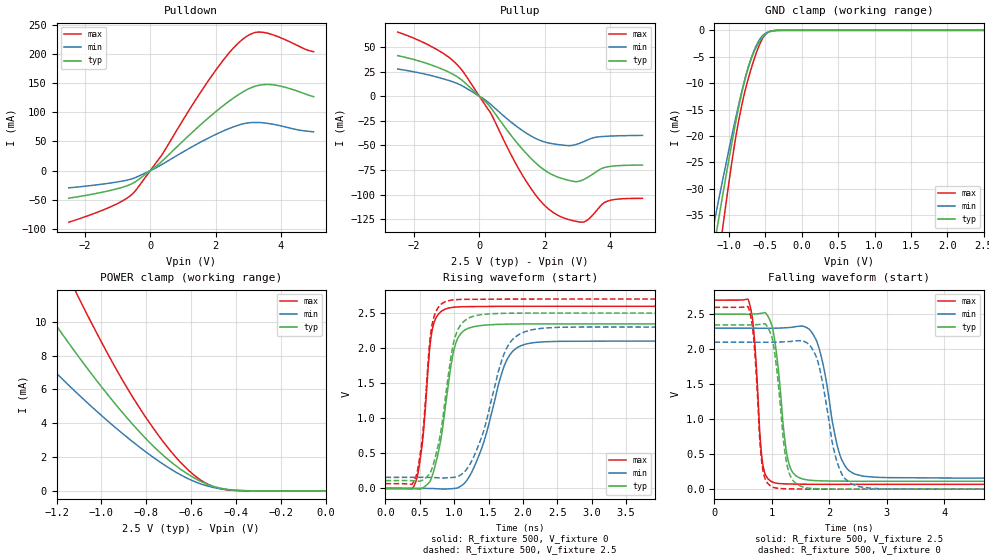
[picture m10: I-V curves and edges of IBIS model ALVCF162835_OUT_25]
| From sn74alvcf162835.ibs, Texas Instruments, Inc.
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[Model]   ALVCF162835_OUT_25
Model_type  3-state
Enable   Active-Low
Vref =   0
Rref =   500
Cref =   30p
Vmeas =   1.25
| variable   typ   min   max
C_comp   2.98pF   2.69pF   3.33pF
| C_pullup   3.41pF   2.52pF   4.48pF
| C_pulldown   2.44pF   2.04pF   2.92pF
| C_tri-state   2.98pF   2.69pF   3.33pF
[Temperature Range]   40   100   -40
| Ambient temperature   25   85   -40
[Voltage range]   2.5   2.3   2.7
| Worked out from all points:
|   slope of the pulldown table from 0 to 0.375 V, typ, clamps not added: 22 ohm
|   slope of the pullup table from 0 to 0.375 V, typ, clamps not added: 29.3 ohm
|   GND clamp passes 1 mA (typ) near -0.52 V on its own axis
|   POWER clamp passes 1 mA (typ) near -0.62 V on its own axis
|   rising waveform, R_fixture 500, V_fixture 0: 20-80 % time 217ps typ, 366ps min, 133ps max; typ from 0 V to 2.35 V
|   falling waveform, R_fixture 500, V_fixture 2.5: 20-80 % time 177ps typ, 283ps min, 116ps max; typ from 2.5 V to 0.112 V
|   rising waveform, R_fixture 500, V_fixture 2.5: 20-80 % time 219ps typ, 366ps min, 134ps max; typ from 0.112 V to 2.5 V
|   falling waveform, R_fixture 500, V_fixture 0: 20-80 % time 177ps typ, 281ps min, 117ps max; typ from 2.35 V to 0 V
[GND Clamp]
| ALVCF162835_OUT_25
|   Voltage   I(typ)   I(min)   I(max)
-2.5V     -156.5mA   -133.7mA   -196.4mA
-1.22V    -42.15mA   -37.53mA   -51.39mA
-1.16V    -37.17mA   -33.34mA   -45.01mA
-1.08V    -30.65mA   -27.85mA   -36.68mA
-925mV    -18.66mA   -17.64mA   -21.71mA
-800mV    -10.4mA    -10.2mA    -12.64mA
-715mV    -6.256mA   -6.058mA   -8.169mA
-645mV    -3.755mA   -3.482mA   -5.072mA
-560mV    -1.73mA    -1.371mA   -2.101mA
-485mV    -620.5uA   -458.2uA   -582.7uA
-295mV    -6.427uA   -8.451uA   -1.684uA
2.5V      1.046nA    413.3nA    70.04pA
[POWER Clamp]
| ALVCF162835_OUT_25
|   Voltage   I(typ)   I(min)   I(max)
-2.5V     39.5mA     27.67mA    55.72mA
-1.515V   16.12mA    11.35mA    23.37mA
-1.28V    11.3mA     8.018mA    16.39mA
-1.115V   8.181mA    5.861mA    11.8mA
-1.095V   7.82mA     5.611mA    11.26mA
-935mV    5.092mA    3.717mA    7.225mA
-810mV    3.206mA    2.388mA    4.506mA
-690mV    1.714mA    1.285mA    2.335mA
-575mV    685.4uA    501.9uA    806.4uA
-505mV    287.7uA    216.5uA    272.5uA
-430mV    75.11uA    63.49uA    49.86uA
-31.15fV  1.046nA    2.588nA    84.19pA
[Pulldown]
| ALVCF162835_OUT_25
|   Voltage   I(typ)   I(min)   I(max)
-2.5V     -47.43mA   -29.66mA   -88.64mA
-1.18V    -33.52mA   -21.01mA   -61.26mA
-515mV    -21.1mA    -13.25mA   -38.15mA
355mV     16mA       10.5mA     27.2mA
1.3V      66.49mA    41.5mA     113.8mA
1.985V    100.3mA    61.58mA    170.9mA
2.49V     122.4mA    73.87mA    207.1mA
2.915V    137.7mA    81.18mA    229.1mA
3.22V     144.9mA    82.63mA    237.2mA
3.55V     147.8mA    81.35mA    236.4mA
4.08V     143.7mA    75.67mA    225.9mA
5V        126.9mA    66.5mA     204.1mA
[Pullup]
| ALVCF162835_OUT_25
|   Voltage   I(typ)   I(min)   I(max)
-2.5V     41.29mA    27.67mA    65.23mA
-1.29V    29.55mA    19.42mA    47.27mA
-595mV    17.89mA    11.75mA    29.04mA
355mV     -11.88mA   -8.484mA   -17.65mA
995mV     -40.82mA   -26.92mA   -61.01mA
1.45V     -58.65mA   -37.79mA   -87.25mA
1.875V    -72.13mA   -45.12mA   -106.6mA
2.26V     -80.25mA   -48.44mA   -118.2mA
2.895V    -86.68mA   -49.71mA   -126.8mA
3.18V     -85mA      -46.42mA   -128.1mA
3.905V    -71.96mA   -40.73mA   -107mA
5V        -70.04mA   -39.87mA   -103.9mA
[Ramp]
| ALVCF162835_OUT_25
| variable   typ   min   max
dV/dt_r   1.41/2.22E-10   1.27/3.69E-10   1.56/1.36E-10
dV/dt_f   1.45/1.91E-10   1.30/2.97E-10   1.59/1.23E-10
R_load = 500
[Rising Waveform]
| ALVCF162835_OUT_25
R_fixture =   500
C_fixture =   0
L_fixture =   0
V_fixture =   0
V_fixture_min = 0
V_fixture_max = 0
|   Time   V(typ)   V(min)   V(max)
0s        -1.061uV   -12.24uV   1.243uV
455ps     -6.551mV   978.1uV    138.1mV
540ps     6.592mV    713.7uV    676mV
650ps     102.2mV    -504uV     2.054V
800ps     664.4mV    -7.051mV   2.514V
995ps     1.971V     -822.8uV   2.584V
1.32ns    2.313V     372.5mV    2.593V
1.78ns    2.343V     1.857V     2.596V
2.18ns    2.346V     2.081V     2.597V
24.99ns   2.346V     2.1V       2.597V
[Falling Waveform]
| ALVCF162835_OUT_25
R_fixture =   500
C_fixture =   0
L_fixture =   0
V_fixture =   2.5
V_fixture_min = 2.3
V_fixture_max = 2.7
|   Time   V(typ)   V(min)   V(max)
0s        2.5V       2.3V       2.7V
595ps     2.499V     2.3V       2.692V
685ps     2.502V     2.3V       2.258V
845ps     2.517V     2.299V     340.7mV
1.105ns   1.768V     2.3V       82.5mV
1.365ns   235.9mV    2.315V     72.88mV
1.765ns   121.9mV    2.142V     69.64mV
2.19ns    114.4mV    476mV      68.92mV
2.625ns   112.7mV    182.2mV    68.79mV
24.99ns   112.2mV    157.7mV    68.81mV
[Rising Waveform]
| ALVCF162835_OUT_25
R_fixture =   500
C_fixture =   0
L_fixture =   0
V_fixture =   2.5
V_fixture_min = 2.3
V_fixture_max = 2.7
|   Time   V(typ)   V(min)   V(max)
0s        112.2mV    157.7mV    68.81mV
455ps     105.7mV    158.5mV    208.8mV
540ps     119.5mV    158.2mV    751.3mV
650ps     217mV      156.9mV    2.142V
800ps     778.6mV    150.7mV    2.616V
990ps     2.072V     158.1mV    2.69V
1.32ns    2.465V     531.4mV    2.697V
1.785ns   2.498V     2.038V     2.7V
2.3ns     2.5V       2.286V     2.7V
24.99ns   2.5V       2.3V       2.7V
[Falling Waveform]
| ALVCF162835_OUT_25
R_fixture =   500
C_fixture =   0
L_fixture =   0
V_fixture =   0
V_fixture_min = 0
V_fixture_max = 0
|   Time   V(typ)   V(min)   V(max)
0s        2.346V     2.1V       2.597V
595ps     2.345V     2.1V       2.585V
685ps     2.348V     2.099V     2.136V
840ps     2.358V     2.099V     289.6mV
1.105ns   1.562V     2.101V     12.49mV
1.37ns    120.3mV    2.114V     3.776mV
1.78ns    7.006mV    1.88V      756.6uV
2.22ns    1.647mV    212.9mV    86.26uV
2.695ns   361uV      15.3mV     -13.07uV
24.99ns   10.3uV     14.65uV    4.303uV
